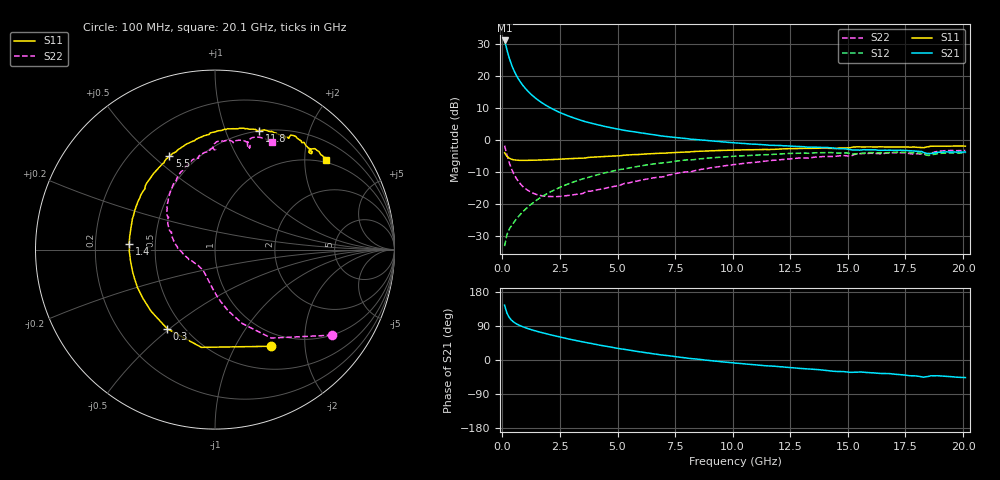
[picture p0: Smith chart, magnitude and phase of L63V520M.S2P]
!  Infineon Technologies AG
! BFR380L3 , PF131585-7, No.6, Th 09.10.01, soldered on pcb-board, measured with PP GSG850
!  Vce=3.5 V,  Ic=20.0 mA
! Common Emitter S-Parameters:  15. November 2001
#  GHz  S  MA  R  50
! f  S11  S21  S12  S22
! GHz  Mag  Ang  Mag  Ang  Mag  Ang  Mag  Ang
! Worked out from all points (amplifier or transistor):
!   201 points, 100 MHz to 20.1 GHz, reference 50 ohm
!   highest |S21| = 31.1 dB at 100 MHz (marker M1)
!   |S21| within 3 dB of that: start of sweep to 203.3 MHz
!   unconditionally stable (mu >= 1): 1.438 GHz to 4.399 GHz
!   at 3.4 GHz: K = 1.02, MAG = 8.4 dB, |S12| = -12.4 dB
!   at 10.1 GHz: K = 0.95, MSG = 2.1 dB, |S12| = -5.2 dB
!   at 20.1 GHz: K = 0.99, MSG = 0.1 dB, |S12| = -4.1 dB
!   S11 on the Smith chart (normalised r, x): 100 MHz: 0.80, -1.41; 300 MHz: 0.41, -0.49; 1.4 GHz: 0.35, +0.03; 5.5 GHz: 0.36, +0.56; 11.8 GHz: 0.50, +1.32; 20.1 GHz: 0.94, +2.52
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0.1  0.6232 -59.8  35.7 144.5  0.02163 63.6  0.8087 -36.1
0.2  0.5499 -98.0  25.52 123.7  0.03255 55.8  0.5837 -57.6
0.3  0.5149 -121.1  19.01 112.3  0.03991 54.1  0.4391 -69.7
0.4  0.4949 -136.0  14.92 105.0  0.04523 54.4  0.3497 -77.8
0.5  0.4848 -146.2  12.22 99.9  0.05088 56.2  0.2913 -83.7
0.6  0.4809 -153.9  10.32 96.0  0.05688 57.7  0.2516 -88.5
0.7  0.4768 -159.9  8.931 92.7  0.06281 59.2  0.2225 -92.7
0.8  0.4755 -164.9  7.868 89.8  0.069 60.3  0.2009 -96.2
0.9  0.4745 -168.9  7.027 87.4  0.07533 61.2  0.1844 -99.5
1.1  0.4753 -175.7  5.8 83.1  0.08808 62.6  0.1624 -105.8
1.4  0.4791 176.0  4.6 77.4  0.1074 63.4  0.1428 -113.7
1.8  0.4828 167.2  3.617 70.9  0.1341 63.2  0.1313 -123.1
2.2  0.4911 159.7  2.999 64.9  0.1602 62.1  0.129 -132.0
2.7  0.5008 151.4  2.484 57.9  0.1933 59.8  0.1323 -141.9
3.5  0.5165 139.7  1.966 47.6  0.245 55.5  0.1447 -154.2
5.5  0.5785 116.0  1.365 26.3  0.361 42.8  0.2112 175.2
6.8  0.6132 103.1  1.162 14.2  0.4299 33.7  0.2601 158.9
10.1  0.6904 78.5  0.8922 -8.1  0.5524 12.3  0.4103 127.0
11.8  0.7073 69.5  0.8143 -16.4  0.592 2.1  0.4774 111.9
13.5  0.7333 60.9  0.7651 -24.6  0.6211 -8.4  0.5293 99.6
16.8  0.7694 48.6  0.6874 -35.9  0.6293 -24.5  0.621 78.4
20.1  0.7929 39.0  0.6429 -46.3  0.6239 -38.3  0.6793 62.1
